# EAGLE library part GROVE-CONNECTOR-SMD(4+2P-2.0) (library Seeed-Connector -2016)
320110030
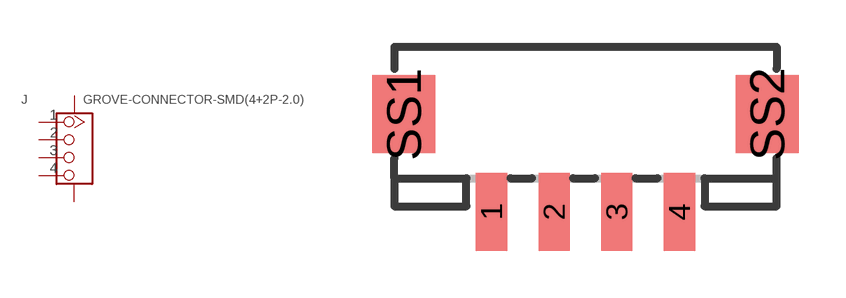
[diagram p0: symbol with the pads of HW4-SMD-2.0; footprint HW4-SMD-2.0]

Designator prefix J

## GROVE-CONNECTOR-SMD(4+2P-2.0) (VALUE: H4P-SMD-2.0)  [HW4-SMD-2.0]
1  1
2  2
3  3
4  4
SS1  SS1
SS2  SS2

## Footprint HW4-SMD-2.0 (pad centres in mm)
smd 1 x 2.5: 1 -3,0; 2 -1,0; 3 1,0; 4 3,0
smd 2 x 2.5: SS1 -5.8,3.123; SS2 5.8,3.123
